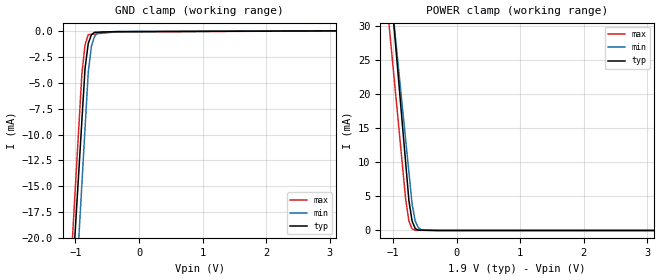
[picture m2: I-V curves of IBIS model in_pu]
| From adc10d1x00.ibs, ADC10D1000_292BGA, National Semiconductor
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[Model] in_pu
Model_type Input
Vinl = 570.000mV
Vinh = 1.33000V
C_comp 1.3pF 1.3pF 1.3pF
| variable typ   min   max
[Voltage Range] 1.90000V 1.80000V 2.00000V
[POWER Clamp Reference] 1.90000V 1.80000V 2.00000V
[GND Clamp Reference] 0.00000V 0.00000V 0.00000V
[Temperature Range]   25   85   -40
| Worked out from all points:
|   GND clamp passes 1 mA (typ) near -0.79 V on its own axis
|   POWER clamp passes 1 mA (typ) near -0.68 V on its own axis
[GND Clamp]
-1.9V     -110.3mA   -122.9mA   -111.5mA
-900mV    -8.695mA   -14.82mA   -4.143mA
-850mV    -3.615mA   -9.42mA    -1.327mA
-800mV    -1.201mA   -4.016mA   -339.1uA
-750mV    -341.5uA   -1.453mA   -307.4uA
-700mV    -109.9uA   -485.4uA   -275.8uA
-650mV    -100.2uA   -181.3uA   -244.1uA
-600mV    -90.62uA   -78.1uA    -212.4uA
-400mV    -52.14uA   -54.26uA   -85.7uA
-350mV    -42.51uA   -48.29uA   -83.97uA
-300mV    -41.46uA   -42.33uA   -82.24uA
3.8V      45.37uA    48.65uA    59.61uA
[POWER Clamp]
-1.9V     130.2mA    116.1mA    112.4mA
-900mV    20.79mA    22.59mA    14.33mA
-800mV    9.855mA    13.25mA    4.522mA
-750mV    4.386mA    8.571mA    1.405mA
-700mV    1.395mA    3.897mA    248.4uA
-650mV    274.2uA    1.353mA    30.51uA
-600mV    42.82uA    393.2uA    26.44uA
-550mV    35.68uA    80uA       22.37uA
3.8V      0A         0A         0A
